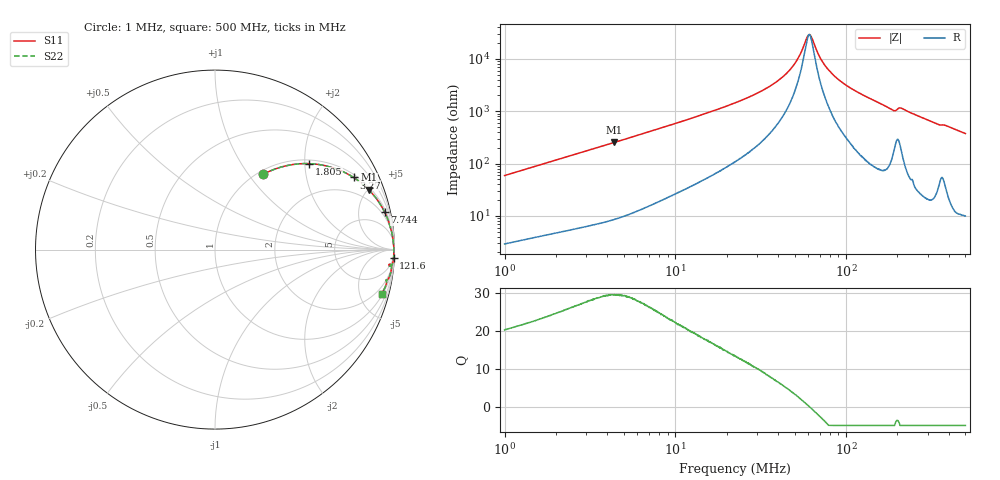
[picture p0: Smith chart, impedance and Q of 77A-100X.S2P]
!s-Parameter Generated by FASTRON Sdn. Bhd.
!FASTRON P/N : 77A-100X
!Keysight Technologies,E4991B,MY54100416,A.01.15
!Date: Mon Mar 16 11:28:53 2026
!Version  : Rev00 Mon Mar 16 11:28:53 2026
!Data & Calibration Information:
!PortZ  Port1:50+j0  Port2:50+j0
!When reading, reference impedance value at option line is always used.
! Remarks : This data is being provided solely for informational purposes.
!Freq	S11	S21	S12	S22
# Hz S dB R 50
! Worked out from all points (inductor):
!   1601 points, 1 MHz to 500 MHz, reference 50 ohm
!   read as one part in series: L = 9.32 uH near 1.032 MHz
!   highest Q = 29.5 at 4.392 MHz (marker M1), where L = 9.16 uH
!   self-resonance near 60.67 MHz
!   S11 on the Smith chart (normalised r, x): 1 MHz: 1.06, +1.18; 1.805 MHz: 1.09, +2.10; 3.27 MHz: 1.13, +3.76; 7.744 MHz: 1.36, +8.96; 121.6 MHz: 4, -43; 500 MHz: 1.20, -7.51
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1000000  -6.06 57.3  -1.48 -29.8  -1.48 -29.8  -6.06 57.3
1804688  -2.98 42.5  -3.40 -45.1  -3.40 -45.1  -2.98 42.5
2820919  -1.53 31.0  -5.76 -56.9  -5.76 -56.9  -1.53 31.0
3269574  -1.20 27.5  -6.70 -60.5  -6.70 -60.5  -1.20 27.5
4392302  -0.73 21.3  -8.79 -66.8  -8.79 -66.8  -0.73 21.3
7744141  -0.28 12.5  -13.32 -75.3  -13.32 -75.3  -0.28 12.5
7957584  -0.27 12.1  -13.55 -75.6  -13.55 -75.6  -0.27 12.1
2.236068e7  -0.07 3.9  -23.25 -81.8  -23.25 -81.8  -0.07 3.9
3.246558e7  -0.04 2.3  -28.03 -81.5  -28.03 -81.5  -0.04 2.3
4.195229e7  -0.04 1.3  -32.80 -78.9  -32.80 -78.9  -0.04 1.3
5.094464e7  -0.03 0.6  -39.00 -71.0  -39.00 -71.0  -0.03 0.6
5.973923e7  -0.03 0.1  -48.81 -18.2  -48.81 -18.2  -0.03 0.1
6.307767e7  -0.03 -0.1  -48.04 32.5  -48.04 32.5  -0.03 -0.1
7.059833e7  -0.03 -0.5  -40.43 69.2  -40.43 69.2  -0.03 -0.5
7.963189e7  -0.03 -0.9  -35.55 78.0  -35.55 78.0  -0.03 -0.9
9.558049e7  -0.03 -1.6  -30.89 82.1  -30.89 82.1  -0.03 -1.6
1.216058e8  -0.04 -2.6  -26.71 83.5  -26.71 83.5  -0.04 -2.6
1.77937e8  -0.09 -4.9  -21.36 80.7  -21.36 80.7  -0.09 -4.9
1.908225e8  -0.18 -5.4  -20.41 74.7  -20.41 74.7  -0.18 -5.4
2.110998e8  -0.14 -4.9  -21.29 76.6  -21.29 76.6  -0.14 -4.9
3.390661e8  -0.20 -9.8  -15.41 77.6  -15.41 77.6  -0.20 -9.8
5e8  -0.35 -14.8  -11.85 73.7  -11.85 73.7  -0.35 -14.8
